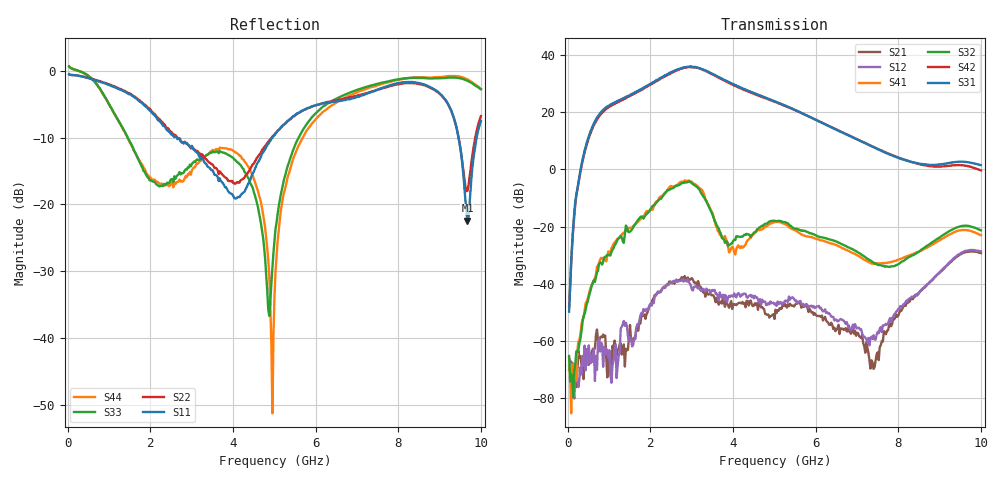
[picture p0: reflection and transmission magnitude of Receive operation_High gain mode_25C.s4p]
! Device:  ADRF5545A
! Description: Dual-Channel, Receiver Front End
! Frequency:  2.4 -  4.2 GHz
! Ports:
!	ANT-CHA	= Port 1
!	ANT-CHB	= Port 2
!  RXOUT-CHA = Port 3
!	RXOUT-CHB = Port 4
! VDD1-CHA, VDD1-CHB, VDD2-CHA, VDD2-CHB, and SWVDD-CHAB = 5 V
! SWCTRL-CHAB = 0 V,  PD-CHAB = 0 V,BP-CHA=BP-CHB=0V
! Temp=25C
! Data:  Data was collected using a calibrated 4 port network analyzer and de-embedded using AtaiTec's In Situ De-Embedding.
! Note:  Analog Devices supplies this data as a sample of measured data
!  for this product.  Your particular data for this product may vary.
!  Data was taken at 25 degrees C.
!  Analog Devices reserves the right to change this data at anytime.
!Correction: S11(Full 4 Port(1,2,3,4))
!S12(Full 4 Port(1,2,3,4))
!S13(Full 4 Port(1,2,3,4))
!S14(Full 4 Port(1,2,3,4))
!S21(Full 4 Port(1,2,3,4))
!S22(Full 4 Port(1,2,3,4))
!S23(Full 4 Port(1,2,3,4))
!S24(Full 4 Port(1,2,3,4))
!S31(Full 4 Port(1,2,3,4))
!S32(Full 4 Port(1,2,3,4))
!S33(Full 4 Port(1,2,3,4))
!S34(Full 4 Port(1,2,3,4))
!S41(Full 4 Port(1,2,3,4))
!S42(Full 4 Port(1,2,3,4))
!S43(Full 4 Port(1,2,3,4))
!S44(Full 4 Port(1,2,3,4))
!S4P File: Measurements: <S11,S12,S13,S14>,
!<S21,S22,S23,S24>,
!<S31,S32,S33,S34>,
!<S41,S42,S43,S44>:
# Hz S  dB  R 50
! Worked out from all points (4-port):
!   400 points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, 34.98 MHz to 10 GHz, reference 50 ohm
!   strongest paths, dB at 34.98 MHz, 2.532 GHz, 5.03 GHz, 7.527 GHz, 10 GHz:
!     S31: -49.7, 34.3, 23.8, 7.0, 1.5
!     S42: -47.8, 33.9, 23.6, 7.0, -0.3
!     S32: -65.3, -6.6, -18.0, -33.4, -21.3
!     S41: -68.8, -6.0, -18.4, -32.9, -23.0
!     S12: -66.1, -39.7, -46.9, -57.4, -28.6
!     S21: -70.1, -39.9, -49.1, -66.8, -29.3
!   lowest |S11| = -22.5 dB at 9.675 GHz (marker M1), VSWR 1.16, Z = 44.1 + j3.87 ohm
!   |S11| at or under -10 dB: 2.637 GHz to 4.952 GHz (2.315 GHz wide, 61 % of centre); 9.459 GHz to 9.898 GHz (439 MHz wide, 4.54 % of centre)
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3.4975e7  -0.48 -10.3  -66.05 62.6  -63.28 -175.8  -64.74 106.5
          -70.09 -107.5  -0.53 -10.1  -60.73 129.0  -64.91 -146.2
          -49.75 -91.7  -65.32 129.0  0.65 -10.0  -70.13 -29.8
          -68.85 15.2  -47.85 -108.2  -76.38 122.3  0.71 -10.0
1.9081e9  -5.41 -131.4  -48.79 -172.6  -60.89 108.7  -80.54 -142.3
          -50.65 178.9  -5.29 -131.2  -71.79 111.4  -59.35 105.0
          29.24 -51.1  -15.65 -51.2  -15.69 138.3  -52.98 -90.1
          -14.60 -53.7  28.94 -48.7  -53.64 -83.0  -15.37 133.4
2.882125e9  -10.77 85.4  -39.24 53.3  -57.67 37.7  -77.24 149.3
            -38.20 51.4  -10.89 91.8  -89.21 68.5  -56.46 29.6
            35.98 177.4  -4.54 93.0  -14.78 8.1  -48.11 145.3
            -3.95 94.6  35.69 -179.7  -48.55 148.8  -15.94 6.3
3.3067e9  -13.67 4.3  -42.13 31.8  -58.46 20.3  -69.57 102.2
          -42.59 4.9  -13.01 11.2  -76.92 138.0  -58.25 25.7
          34.87 108.6  -9.93 -45.8  -12.81 -18.7  -50.47 111.8
          -8.95 -48.9  34.74 110.1  -49.45 122.2  -12.90 -29.1
3.95605e9  -18.37 -36.4  -44.11 12.9  -56.79 -1.9  -76.86 85.0
           -46.05 2.4  -16.54 -16.3  -74.70 85.2  -57.27 -4.8
           30.25 30.5  -25.96 107.3  -12.85 -40.2  -49.35 99.3
           -27.61 71.7  29.94 32.3  -53.07 112.8  -11.81 -46.7
9.675325e9  -22.45 144.6  -28.35 -113.5  -62.37 104.2  -61.03 45.6
            -28.83 -121.3  -17.95 149.5  -59.46 41.1  -63.43 70.3
            2.57 -14.0  -19.72 -67.6  -1.49 113.2  -59.58 100.8
            -21.26 -67.2  1.23 -14.9  -62.28 104.8  -1.27 105.8
1e10  -7.50 -146.8  -28.62 -169.7  -61.63 143.7  -63.31 42.6
      -29.30 -178.1  -6.78 -158.5  -64.03 59.7  -67.79 105.7
      1.52 -52.6  -21.30 -127.9  -2.76 115.0  -59.06 102.7
      -23.02 -125.6  -0.31 -52.0  -61.76 99.6  -2.70 109.0
